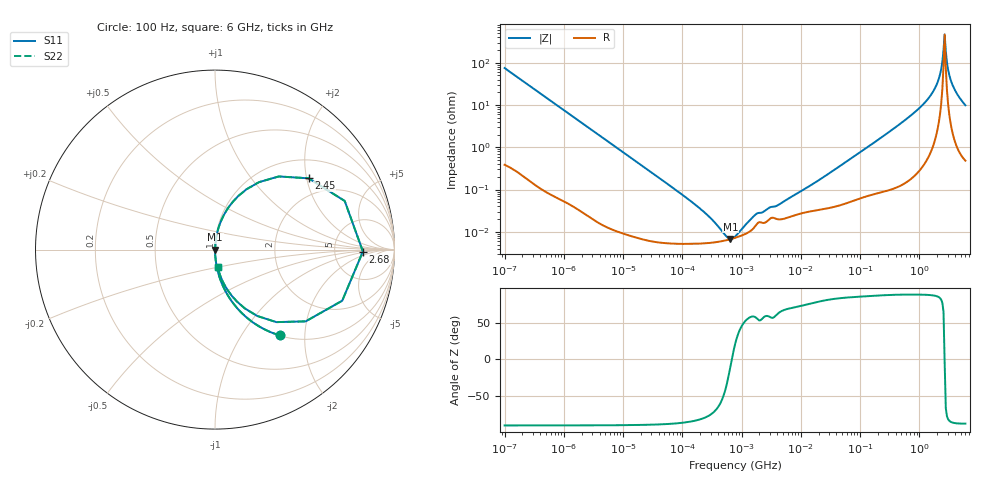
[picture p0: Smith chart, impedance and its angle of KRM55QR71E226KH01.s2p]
!Murata Part Number: KRM55QR71E226KH01
!These Parameters are Measured in Series Mode Connection
!Data Generated on Jan 08, 2026
!  o--ll--o
!Port1  Port2
!  o------o
!Operation Temp=25[degC], DC Bias Voltage=0[V]
!Freq. Start=100[Hz] Stop=6[GHz] 401[Steps]
# Hz S RI R 50
!Freq.(Hz) S11(Real) S11(Imag) S21(Real) S21(Imag) S12(Real) S12(Imag) S22(Real) S22(Imag)
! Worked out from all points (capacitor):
!   401 points, 100 Hz to 6 GHz, reference 50 ohm
!   read as one part in series: C = 21.1 uF near 109 Hz
!   lowest |Z| = 6.8 mohm at 647.6 kHz (marker M1)
!   series resonance near 683.4 kHz, so ESL is about 2.6 nH
!   S11 on the Smith chart (normalised r, x): 100 Hz: 1.01, -1.50; 2.45 GHz: 1.47, +2.05; 2.68 GHz: 10, -1; 6 GHz: 1.01, -0.20
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100  0.3614 -0.4779  0.6386 0.4779  0.6386 0.4779  0.3614 -0.4779
306  0.0584 -0.2317  0.9416 0.2317  0.9416 0.2317  0.0584 -0.2317
2008  0.00172 -0.0378  0.9983 0.0378  0.9983 0.0378  0.00172 -0.0378
40335  5.95e-05 -0.0019  0.9999 0.0019  0.9999 0.0019  5.95e-05 -0.0019
202169  5.28e-05 -0.000345  0.9999 0.000345  0.9999 0.000345  5.28e-05 -0.000345
473344  6.04e-05 -8.19e-05  0.9999 8.19e-05  0.9999 8.19e-05  6.04e-05 -8.19e-05
647581  6.7e-05 -1.16e-05  0.9999 1.16e-05  0.9999 1.16e-05  6.7e-05 -1.16e-05
774597  7.2e-05 2.66e-05  0.9999 -2.66e-05  0.9999 -2.66e-05  7.2e-05 2.66e-05
968953  8.02e-05 7.46e-05  0.9999 -7.46e-05  0.9999 -7.46e-05  8.02e-05 7.46e-05
1813585  0.000153 0.000224  0.9998 -0.000224  0.9998 -0.000224  0.000153 0.000224
4060267  0.000199 0.000373  0.9998 -0.000373  0.9998 -0.000373  0.000199 0.000373
1.555665e7  0.000312 0.00129  0.9997 -0.00129  0.9997 -0.00129  0.000312 0.00129
3.124326e8  0.00151 0.0233  0.9985 -0.0233  0.9985 -0.0233  0.00151 0.0233
9.569533e8  0.00885 0.0789  0.9911 -0.0789  0.9911 -0.0789  0.00885 0.0789
1.712697e9  0.051 0.1956  0.949 -0.1956  0.949 -0.1956  0.051 0.1956
2.142435e9  0.1752 0.3359  0.8248 -0.3359  0.8248 -0.3359  0.1752 0.3359
2.450438e9  0.5214 0.3971  0.4786 -0.3971  0.4786 -0.3971  0.5214 0.3971
2.679998e9  0.824 -0.0107  0.176 0.0107  0.176 0.0107  0.824 -0.0107
2.931063e9  0.5054 -0.3998  0.4946 0.3998  0.4946 0.3998  0.5054 -0.3998
3.065283e9  0.342 -0.404  0.658 0.404  0.658 0.404  0.342 -0.404
3.666503e9  0.094 -0.2579  0.906 0.2579  0.906 0.2579  0.094 -0.2579
6e9  0.0143 -0.0965  0.9857 0.0965  0.9857 0.0965  0.0143 -0.0965
